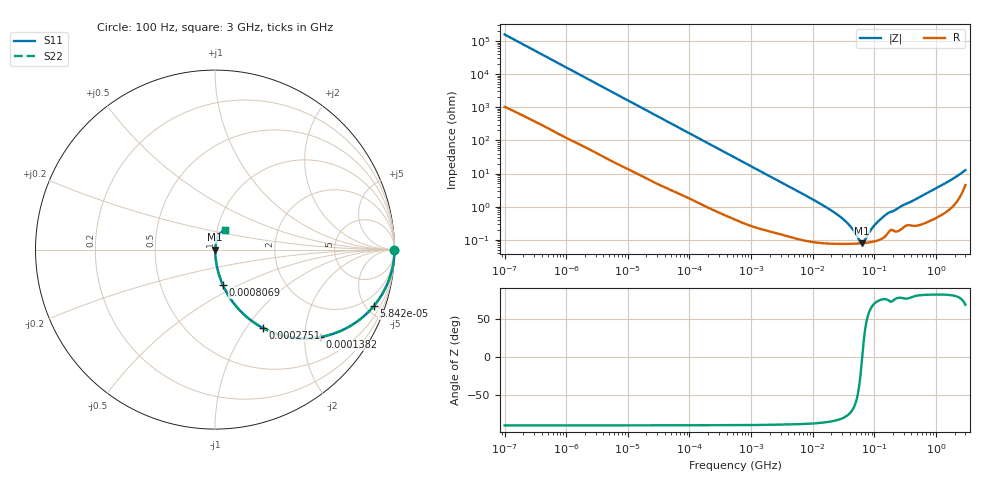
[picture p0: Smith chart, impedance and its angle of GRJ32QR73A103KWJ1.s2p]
!Murata Part Number: GRJ32QR73A103KWJ1
!These Parameters are Measured in Series Mode Connection
!Data Generated on Jun 19, 2026
!  o--ll--o
!Port1  Port2
!  o------o
!Operation Temp=25[degC], DC Bias Voltage=0[V]
!Freq. Start=100[Hz] Stop=3[GHz] 401[Steps]
# Hz S RI R 50
!Freq.(Hz) S11(Real) S11(Imag) S21(Real) S21(Imag) S12(Real) S12(Imag) S22(Real) S22(Imag)
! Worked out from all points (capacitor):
!   401 points, 100 Hz to 3 GHz, reference 50 ohm
!   read as one part in series: C = 10.1 nF near 109 Hz
!   lowest |Z| = 78.9 mohm at 62.34 MHz (marker M1)
!   series resonance near 63.35 MHz, so ESL is about 630 pH
!   S11 on the Smith chart (normalised r, x): 100 Hz: open; 58.42 kHz: 1.06, -5.58; 138.2 kHz: 1.03, -2.37; 275.1 kHz: 1.01, -1.20; 806.9 kHz: 1.01, -0.41; 3 GHz: 1.09, +0.24
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100  1 -0.000633  4.5e-06 0.000633  4.5e-06 0.000633  1 -0.000633
1788  0.9998 -0.0112  0.000212 0.0112  0.000212 0.0112  0.9998 -0.0112
10003  0.9957 -0.0617  0.00434 0.0617  0.00434 0.0617  0.9957 -0.0617
31977  0.9611 -0.1888  0.0389 0.1888  0.0389 0.1888  0.9611 -0.1888
58416  0.8838 -0.3155  0.1162 0.3155  0.1162 0.3155  0.8838 -0.3155
89839  0.7657 -0.4183  0.2343 0.4183  0.2343 0.4183  0.7657 -0.4183
138163  0.584 -0.4875  0.416 0.4875  0.416 0.4875  0.584 -0.4875
275091  0.2664 -0.4362  0.7336 0.4362  0.7336 0.4362  0.2664 -0.4362
547723  0.0868 -0.2748  0.9132 0.2748  0.9132 0.2748  0.0868 -0.2748
806856  0.0432 -0.1962  0.9568 0.1962  0.9568 0.1962  0.0432 -0.1962
2266852  0.00705 -0.073  0.9929 0.073  0.9929 0.073  0.00705 -0.073
9794414  0.00114 -0.0169  0.9989 0.0169  0.9989 0.0169  0.00114 -0.0169
3.131008e7  0.000765 -0.0041  0.9992 0.0041  0.9992 0.0041  0.000765 -0.0041
4.231884e7  0.000759 -0.00222  0.9992 0.00222  0.9992 0.00222  0.000759 -0.00222
5.719833e7  0.000775 -0.000549  0.9992 0.000549  0.9992 0.000549  0.000775 -0.000549
6.234031e7  0.000784 -8.55e-05  0.9992 8.55e-05  0.9992 8.55e-05  0.000784 -8.55e-05
6.794454e7  0.000795 0.000378  0.9992 -0.000378  0.9992 -0.000378  0.000795 0.000378
8.79653e7  0.000852 0.0018  0.9991 -0.0018  0.9991 -0.0018  0.000852 0.0018
1.090876e8  0.000939 0.00309  0.9991 -0.00309  0.9991 -0.00309  0.000939 0.00309
1.751444e8  0.00185 0.00645  0.9981 -0.00645  0.9981 -0.00645  0.00185 0.00645
1.214989e9  0.00731 0.0427  0.9927 -0.0427  0.9927 -0.0427  0.00731 0.0427
3e9  0.0549 0.1072  0.9451 -0.1072  0.9451 -0.1072  0.0549 0.1072
